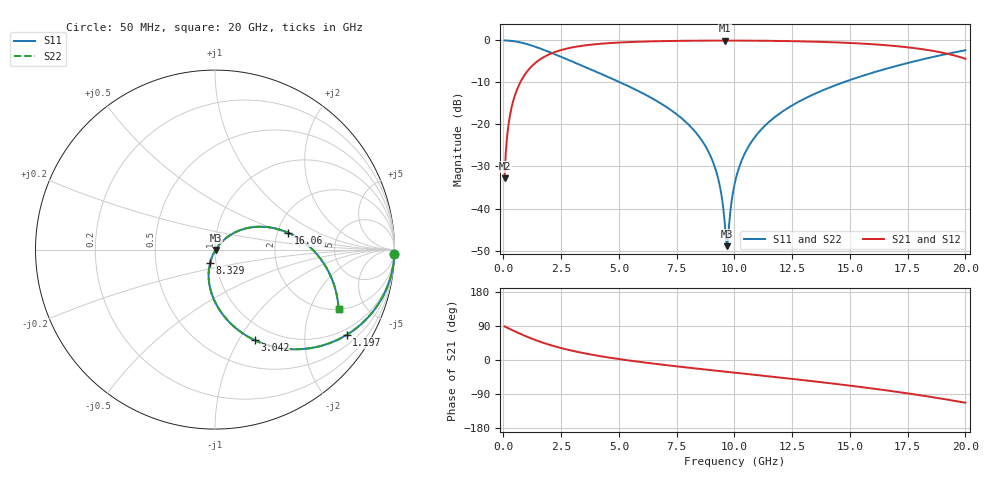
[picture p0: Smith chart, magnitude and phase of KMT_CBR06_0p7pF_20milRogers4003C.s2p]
! Data measured by Modelithics Inc. support@modelithics.com 813-866-6335
! KEMET CBR0603 0.7pF, Pad Width= 0.851mm, Pad Length= 0.64mm, Pad Gap= 0.62mm, 20mil Rogers 4003C substrate Data, January 2022
# hz S ma R 50
! 2 Port Network Data from SP1.SP block
! freq  magS11  angS11  magS21  angS21  magS12  angS12  magS22  angS22
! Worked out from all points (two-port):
!   401 points, 50 MHz to 20 GHz, reference 50 ohm
!   highest |S21| = -0.03 dB at 9.576 GHz (marker M1); lowest = -32.8 dB at 50 MHz (marker M2)
!   |S21| within 3 dB of the highest: 2.1 GHz to 19.11 GHz (17.01 GHz wide, 160 % of centre)
!   lowest |S11| = -49.0 dB at 9.676 GHz (marker M3), VSWR 1.01, Z = 50.3 - j0.199 ohm
!   |S11| at or under -10 dB: 5.063 GHz to 14.7 GHz (9.637 GHz wide, 97.5 % of centre)
!   |S22| runs from -49.0 to 0.0 dB; largest |S21 - S12| = 0
!   S11 on the Smith chart (normalised r, x): 50 MHz: 1, -78; 1.197 GHz: 0.80, -3.21; 3.042 GHz: 0.81, -1.17; 8.329 GHz: 0.94, -0.14; 16.06 GHz: 2.30, +0.52; 20 GHz: 2.00, -3.20
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5e7  0.9997 -1.5  0.02286 88.5  0.02286 88.5  0.9997 -1.5
2.495e8  0.9935 -7.3  0.1134 82.7  0.1134 82.7  0.9935 -7.3
4.49e8  0.9794 -13.1  0.2015 76.9  0.2015 76.9  0.9794 -13.1
1.197125e9  0.8743 -32.9  0.4844 57.0  0.4844 57.0  0.8743 -32.9
1.94525e9  0.7358 -48.9  0.6758 41.0  0.6758 41.0  0.7358 -48.9
3.0425e9  0.5515 -66.3  0.8322 23.5  0.8322 23.5  0.5515 -66.3
3.391625e9  0.502 -70.7  0.8628 19.1  0.8628 19.1  0.502 -70.7
4.838e9  0.3373 -85.7  0.9389 3.9  0.9389 3.9  0.3373 -85.7
6.73325e9  0.1836 -100.4  0.98 -11.3  0.98 -11.3  0.1836 -100.4
8.32925e9  0.08024 -110.1  0.9933 -22.4  0.9933 -22.4  0.08024 -110.1
9.177125e9  0.02963 -111.4  0.9958 -28.0  0.9958 -28.0  0.02963 -111.4
9.4265e9  0.01517 -106.4  0.9961 -29.6  0.9961 -29.6  0.01517 -106.4
9.576125e9  0.006953 -90.1  0.9961 -30.6  0.9961 -30.6  0.006953 -90.1
9.675875e9  0.003562 -33.7  0.9961 -31.3  0.9961 -31.3  0.003562 -33.7
9.775625e9  0.00672 25.8  0.996 -31.9  0.996 -31.9  0.00672 25.8
1.0025e10  0.02058 46.2  0.9958 -33.5  0.9958 -33.5  0.02058 46.2
1.0424e10  0.04375 48.9  0.9949 -36.1  0.9949 -36.1  0.04375 48.9
1.107238e10  0.08186 46.8  0.9922 -40.4  0.9922 -40.4  0.08186 46.8
1.336662e10  0.2244 32.8  0.9686 -55.8  0.9686 -55.8  0.2244 32.8
1.605988e10  0.4191 12.9  0.8985 -75.9  0.8985 -75.9  0.4191 12.9
1.670825e10  0.4716 7.5  0.8708 -81.2  0.8708 -81.2  0.4716 7.5
2e10  0.7643 -25.8  0.6052 -112.8  0.6052 -112.8  0.7643 -25.8
